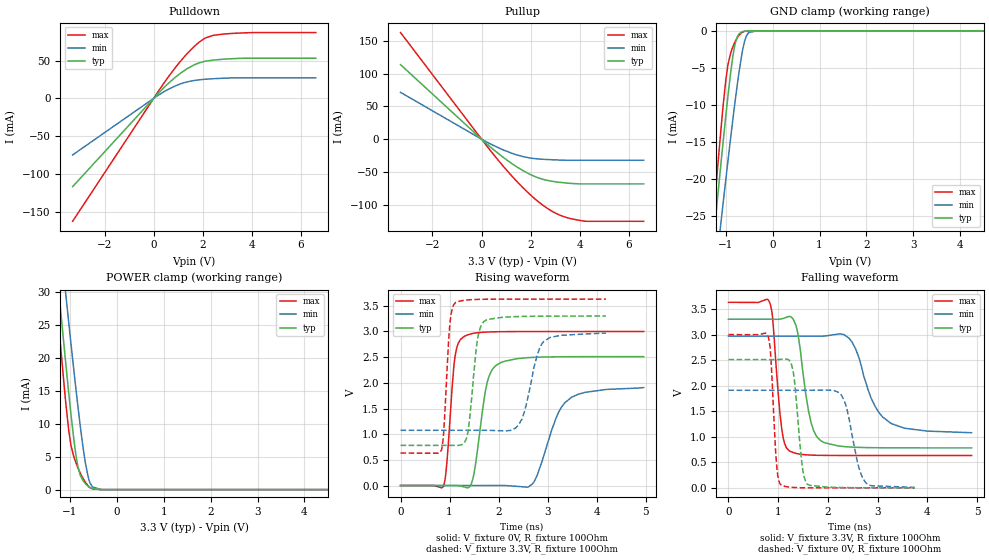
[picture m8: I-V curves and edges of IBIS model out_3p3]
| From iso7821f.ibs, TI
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|   out_3p3 Model
[Model]   out_3p3
Model_type   3-state
Polarity   Non-Inverting
Vmeas = 1.65
Vref = 0
Cref = 15pF
Rref = 150
|   typ   min   max
|   (nom PVT)   (fast PVT)   (slow PVT)
C_comp   9.270e-13   8.382e-13   1.039e-12
| Where nom  PVT is Nominal Process, 3.3V, 27C
|   Fast PVT is Strong Process,  3.63V, -55C
|   Slow PVT is Weak Process,   2.97V, 150C
[Voltage Range]   3.3   2.97   3.63
|Junction Temperature
[Temperature Range]   27   150   -55
[Pullup Reference]   3.3   2.97   3.63
[Pulldown Reference]   0   0   0
[Power Clamp Reference]   3.3   2.97   3.63
[GND Clamp Reference]   0   0   0
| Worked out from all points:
|   slope of the pulldown table from 0 to 0.495 V, typ, clamps not added: 29.7 ohm
|   slope of the pullup table from 0 to 0.495 V, typ, clamps not added: 30.6 ohm
|   GND clamp passes 1 mA (typ) near -0.76 V on its own axis
|   POWER clamp passes 1 mA (typ) near -0.68 V on its own axis
|   falling waveform, V_fixture 3.3V, R_fixture 100Ohm: 20-80 % time 229ps typ, 434ps min, 150ps max; typ from 3.3 V to 0.782 V
|   rising waveform, V_fixture 0V, R_fixture 100Ohm: 20-80 % time 225ps typ, 428ps min, 139ps max; typ from 0 V to 2.51 V
|   rising waveform, V_fixture 3.3V, R_fixture 100Ohm: 20-80 % time 155ps typ, 276ps min, 104ps max; typ from 0.782 V to 3.3 V
|   falling waveform, V_fixture 0V, R_fixture 100Ohm: 20-80 % time 138ps typ, 240ps min, 94.9ps max; typ from 2.51 V to 0 V
[Pulldown]
|   Voltage   I(typ)   I(min)   I(max)
-3.3V     -116.8mA   -74.8mA    -162.6mA
67.98mV   2.426mA    1.528mA    3.39mA
463mV     15.67mA    9.587mA    22.3mA
860mV     27.32mA    16.13mA    39.76mA
1.256V    37mA       20.88mA    55.31mA
1.633V    44.06mA    23.59mA    68.06mA
1.858V    47.02mA    24.56mA    74.44mA
2.123V    49.2mA     25.37mA    80.1mA
2.414V    50.61mA    26.01mA    83.21mA
2.867V    51.88mA    26.71mA    85.18mA
3.97V     53.09mA    27.18mA    86.97mA
6.6V      53.09mA    27.18mA    87.05mA
[GND Clamp]
|   Voltage   I(typ)   I(min)   I(max)
-3.3V     -170.3mA   -157.8mA   -194.4mA
-1.317V   -32.1mA    -38.42mA   -29.69mA
-1.236V   -26.73mA   -33.72mA   -23.39mA
-1.158V   -21.65mA   -29.24mA   -17.5mA
-1.073V   -16.16mA   -24.35mA   -11.34mA
-953.7mV  -8.946mA   -17.72mA   -4.696mA
-879.4mV  -4.954mA   -13.71mA   -2.735mA
-798.6mV  -1.751mA   -9.533mA   -1.459mA
-656.7mV  -152.7uA   -3.229mA   -238.9uA
-558.7mV  -21.74uA   -692.2uA   -27.8uA
-330mV    -65.89nA   -2.179uA   -17.08nA
6.6V      0A         0A         0A
[Pullup]
|   Voltage   I(typ)   I(min)   I(max)
-3.3V     113.7mA    71.42mA    162.6mA
0V        0A         0A         0A
742.2mV   -23.69mA   -14.11mA   -35.04mA
1.223V    -37.05mA   -21.36mA   -55.86mA
1.648V    -47.2mA    -26.21mA   -72.73mA
2.043V    -54.93mA   -29.12mA   -86.88mA
2.406V    -60.25mA   -30.47mA   -98.28mA
2.824V    -63.99mA   -31.34mA   -109.1mA
3.209V    -65.98mA   -31.95mA   -116.3mA
3.994V    -68.26mA   -32.19mA   -124mA
4.279V    -68.26mA   -32.19mA   -125.3mA
6.6V      -68.26mA   -32.19mA   -125.3mA
[POWER Clamp]
|   Voltage   I(typ)   I(min)   I(max)
-3.3V     196.1mA    190mA      211.9mA
-1.367V   40.17mA    49.19mA    36mA
-1.274V   33.06mA    42.63mA    28.11mA
-1.198V   27.34mA    37.33mA    21.84mA
-1.081V   18.74mA    29.25mA    12.78mA
-973.2mV  11.25mA    21.94mA    6.628mA
-891mV    6.299mA    16.58mA    4.476mA
-825mV    3.399mA    12.45mA    3.258mA
-668.6mV  913.7uA    4.04mA     1.1mA
-592mV    415.6uA    1.476mA    435.3uA
-517.1mV  136.9uA    396.6uA    105.4uA
6.6V      0A         0A         0A
[Ramp]
R_load = 100
|   typ   min   max
dV/dt_r   1.50593/2.25209e-10   1.14448/4.27706e-10   1.79944/1.3814e-10
dV/dt_f   1.51075/2.27699e-10   1.13579/4.29653e-10   1.79824/1.49241e-10
[Falling Waveform]
V_fixture = 3.3V
V_fixture_min = 2.97V
V_fixture_max = 3.63V
R_fixture = 100Ohm
|   Time   V(typ)   V(min)   V(max)
0s        3.3V       2.97V      3.63V
828ps     3.3V       2.97V      3.63V
1.07ns    3.308V     2.97V      1.165V
1.218ns   3.355V     2.97V      729.6mV
1.378ns   3.102V     2.97V      670.1mV
1.66ns    1.286V     2.969V     641mV
1.852ns   926.1mV    2.969V     636.2mV
2.424ns   800.9mV    2.929V     633.2mV
3.274ns   783.5mV    1.258V     633mV
4.89ns    782.1mV    1.079V     632.9mV
[Rising Waveform]
V_fixture = 0V
V_fixture_min = 0V
V_fixture_max = 0V
R_fixture = 100Ohm
|   Time   V(typ)   V(min)   V(max)
0s        3.012nV    81.93nV    1.808nV
874ps     -58.34uV   -35.64nV   -21.56mV
1.108ns   1.239mV    3.56uV     2.486V
1.292ns   -25.13mV   605.8nV    2.9V
1.468ns   102.9mV    -38.81uV   2.96V
1.73ns    1.836V     108.4uV    2.988V
1.954ns   2.344V     1.266mV    2.995V
2.688ns   2.495V     30.32mV    2.999V
3.492ns   2.509V     1.72V      2.999V
4.96ns    2.51V      1.907V     2.999V
[Rising Waveform]
V_fixture = 3.3V
V_fixture_min = 2.97V
V_fixture_max = 3.63V
R_fixture = 100Ohm
|   Time   V(typ)   V(min)   V(max)
0s        782mV      1.075V     632.8mV
838ps     782.1mV    1.075V     696.1mV
1.008ns   782.3mV    1.075V     3.155V
1.124ns   780.6mV    1.075V     3.564V
1.362ns   968.5mV    1.075V     3.614V
1.546ns   2.689V     1.075V     3.624V
1.702ns   3.195V     1.076V     3.627V
2.408ns   3.291V     1.183V     3.63V
2.914ns   3.298V     2.799V     3.63V
4.19ns    3.3V       2.969V     3.63V
[Falling Waveform]
V_fixture = 0V
V_fixture_min = 0V
V_fixture_max = 0V
R_fixture = 100Ohm
|   Time   V(typ)   V(min)   V(max)
0s        2.51V      1.91V      2.999V
798ps     2.51V      1.91V      2.966V
974ps     2.51V      1.91V      394.1mV
1.074ns   2.517V     1.91V      42.7mV
1.3ns     2.294V     1.91V      8.652mV
1.484ns   423.8mV    1.909V     2.338mV
1.586ns   72.41mV    1.909V     1.139mV
2.282ns   6.595mV    1.796V     26.25uV
2.756ns   1.947mV    106.3mV    3.643uV
3.744ns   225.5uV    9.728mV    72.97nV
